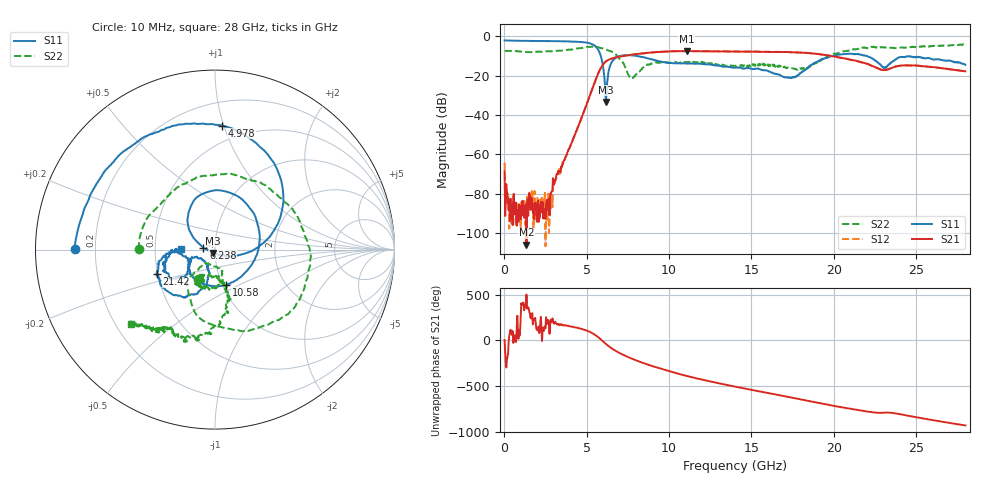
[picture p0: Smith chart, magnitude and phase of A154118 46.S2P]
!  2-Port S-parameters saved by WinCal
! VAR MeasName=S-Parameters (CALIBRATED_DATA) read from VNA (N5230A)
! VAR MeasDate=2015-9-10 14:38:02
! VAR NAME=A154118 46
! VAR FILENAME=A154118 46.S2P
! VAR DATE=2015-9-10 14:38:02
! VAR PHYS_PORTS=1,2
# Hz S DB R 50
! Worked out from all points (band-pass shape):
!   801 points, 10 MHz to 28 GHz, reference 50 ohm
!   highest |S21| = -7.56 dB at 11.07 GHz (marker M1); lowest = -105.7 dB at 1.34 GHz (marker M2)
!   |S21| within 3 dB of the highest: 6.858 GHz to 20.2 GHz (13.34 GHz wide, 98.6 % of centre)
!   lowest |S11| = -33.3 dB at 6.168 GHz (marker M3), VSWR 1.04, Z = 49 - j1.87 ohm
!   |S11| at or under -10 dB: 5.849 GHz to 7.012 GHz (1.162 GHz wide, 18.1 % of centre); 8.049 GHz to 19.89 GHz (11.84 GHz wide, 84.8 % of centre); 21.99 GHz to end of sweep
!   |S22| runs from -21.4 to -4.1 dB; largest |S21 - S12| = 0.0073
!   S11 on the Smith chart (normalised r, x): 10 MHz: 0.12, +0.00; 4.978 GHz: 0.37, +0.99; 6.238 GHz: 0.88, +0.02; 10.58 GHz: 1.05, -0.43; 21.42 GHz: 0.49, -0.16; 28 GHz: 0.68, +0.00
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1e7  -2.15 179.7  -68.35 1.0  -64.14 67.0  -7.50 179.8
1.849375e8  -2.16 177.2  -81.93 178.1  -85.82 23.3  -7.44 174.3
1.339525e9  -2.36 162.3  -105.73 139.8  -85.84 57.5  -8.06 140.9
2.774012e9  -2.50 142.1  -80.07 175.2  -82.51 175.9  -7.66 97.3
4.698325e9  -3.01 98.2  -41.06 123.3  -40.95 123.3  -5.94 11.3
4.978225e9  -3.20 86.5  -34.90 106.8  -34.87 107.1  -5.41 -3.9
5.712962e9  -7.19 31.0  -18.55 30.6  -18.53 30.4  -5.67 -49.4
6.1678e9  -33.31 -117.8  -12.77 -41.8  -12.76 -41.9  -6.68 -76.1
6.237775e9  -23.66 170.5  -12.36 -52.4  -12.34 -52.5  -6.97 -79.7
6.657625e9  -11.68 123.4  -10.98 -105.9  -11.00 -106.1  -8.44 -105.7
7.70725e9  -9.72 74.5  -9.42 160.4  -9.41 160.1  -21.40 -115.4
9.351662e9  -12.56 -6.5  -8.00 55.5  -7.97 55.3  -13.53 -92.8
1.057622e10  -13.78 -72.1  -7.57 -8.1  -7.55 -8.6  -13.63 -106.8
1.106605e10  -13.86 -94.4  -7.56 -30.9  -7.50 -31.3  -13.18 -109.8
1.243056e10  -14.24 -135.8  -7.63 -88.4  -7.58 -89.0  -14.14 -123.4
1.4005e10  -15.98 -152.6  -7.79 -148.0  -7.77 -148.4  -15.10 -120.5
1.73638e10  -20.98 -131.6  -8.09 94.7  -8.11 94.0  -16.22 -112.7
1.869332e10  -14.31 -103.4  -8.72 47.2  -8.73 46.6  -14.02 -76.9
2.142235e10  -9.07 -157.0  -12.62 -43.7  -12.62 -44.2  -6.54 -97.0
2.334666e10  -14.53 -141.7  -16.62 -72.5  -16.65 -73.1  -6.01 -119.0
2.457122e10  -10.18 -157.0  -14.81 -108.4  -14.81 -109.7  -5.57 -123.8
2.8e10  -14.55 179.6  -17.76 146.8  -17.88 146.2  -4.09 -138.2
